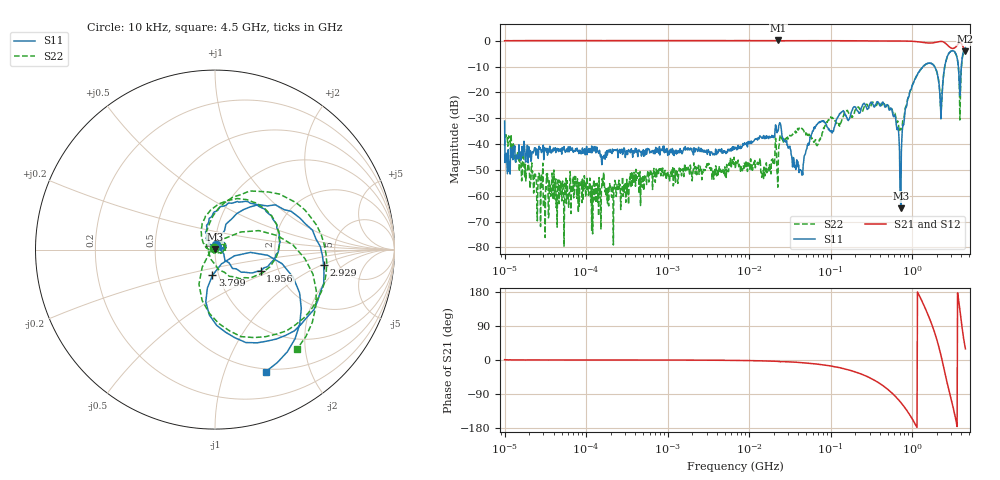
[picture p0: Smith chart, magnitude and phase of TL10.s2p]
!Siglent Technologies,SNA5004A,SNA5XCED5R0097,V1.0.0.2.10.R9
!Date: 2024-11-24 17:21:03
!Data & Calibration Information:
!Freq	S11:F2(ON)	S21:F2(ON)	S12:F2(ON)	S22:F2(ON)
# Hz S DB R 50
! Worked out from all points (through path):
!   1001 points, 10 kHz to 4.5 GHz, reference 50 ohm
!   highest |S21| = 0.11 dB at 22.8 MHz (marker M1); lowest = -4.0 dB at 4.5 GHz (marker M2)
!   group delay of S21, straight-line fit = 427 ps
!   lowest |S11| = -64.8 dB at 727.4 MHz (marker M3), VSWR 1.00, Z = 50 + j0.057 ohm
!   |S11| at or under -10 dB: start of sweep to 1.354 GHz; 1.879 GHz to 2.511 GHz (631.8 MHz wide, 28.8 % of centre); 3.687 GHz to 4.016 GHz (329.8 MHz wide, 8.56 % of centre)
!   |S22| runs from -79.5 to -2.9 dB; largest |S21 - S12| = 0.022
!   S11 on the Smith chart (normalised r, x): 10 kHz: 1.01, +0.06; 1.956 GHz: 1.62, -0.42; 2.929 GHz: 3.84, -1.04; 3.799 GHz: 0.93, -0.27; 4.5 GHz: 0.47, -1.39
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10000  -31.09 81.9  0.01 0.8  -0.02 0.9  -40.76 108.1
10953.99  -46.33 30.9  0.06 0.4  -0.00 0.2  -40.82 70.8
29458.91  -40.86 0.5  0.07 0.2  0.02 0.1  -47.41 73.9
87919.76  -43.73 13.2  0.06 0.0  0.00 -0.1  -54.46 -40.9
772988.4  -43.29 17.9  0.06 -0.1  0.01 -0.2  -51.40 -57.0
6708204  -41.62 62.4  0.05 -1.0  -0.02 -1.2  -47.40 -131.2
1.484063e7  -37.78 98.0  0.05 -2.4  -0.02 -2.5  -50.22 -41.2
2.280385e7  -34.54 118.8  0.11 -3.8  0.04 -3.8  -46.60 97.9
4.259537e7  -50.15 111.9  0.07 -6.8  -0.04 -6.8  -34.21 80.7
5.897837e7  -35.89 45.8  0.03 -9.4  -0.04 -9.4  -37.61 102.0
2.313556e8  -27.66 46.0  -0.03 -36.1  -0.11 -35.9  -26.60 52.2
5.185364e8  -26.59 15.1  -0.09 -80.1  -0.15 -79.8  -25.70 -1.4
7.273824e8  -64.85 95.2  -0.11 -112.2  -0.15 -112.0  -33.90 -111.7
8.727859e8  -23.34 124.8  -0.13 -135.0  -0.19 -134.7  -23.13 152.1
1.240351e9  -11.47 74.3  -0.48 167.6  -0.52 167.9  -11.63 82.2
1.609195e9  -8.60 22.0  -0.89 113.2  -0.94 113.6  -8.66 24.2
1.956171e9  -11.02 -25.2  -0.60 62.0  -0.66 62.6  -10.95 -29.0
2.377963e9  -16.25 66.7  -0.38 -8.9  -0.43 -8.2  -16.30 100.7
2.928576e9  -4.28 -8.0  -2.59 -93.4  -2.61 -92.6  -4.32 3.2
3.379417e9  -4.65 -60.7  -2.57 -149.9  -2.65 -149.2  -4.70 -54.1
3.79945e9  -16.84 -95.6  -0.75 142.8  -0.81 143.6  -18.32 -126.0
4.5e9  -2.66 -67.4  -4.02 29.5  -4.05 30.9  -2.87 -50.5
